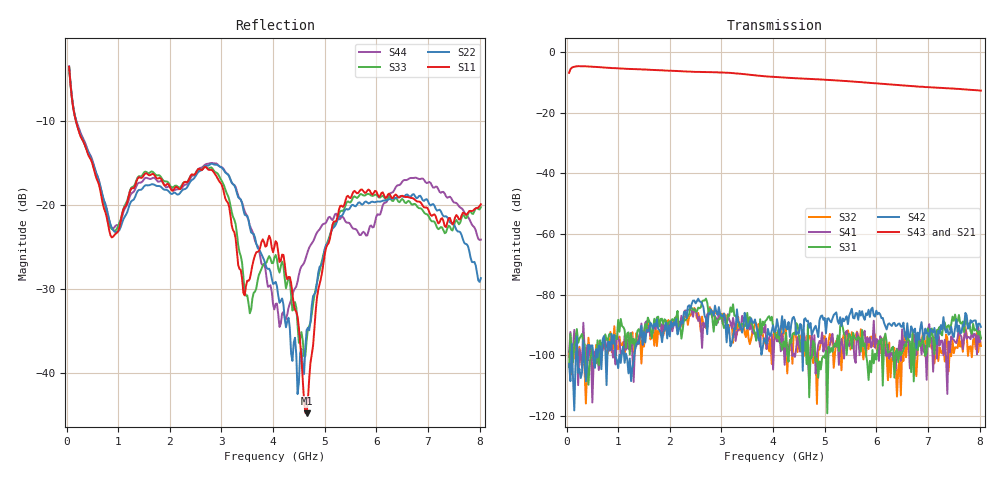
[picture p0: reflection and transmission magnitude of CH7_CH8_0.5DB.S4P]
!Agilent Technologies,E5071C,MY46316741,A.11.02
!Date: Mon Jun 01 10:30:22 2026
!Data & Calibration Information:
!1:CH7 INPUT 2:CH7 OUTPUT 3:CH8 INPUT 4:CH8 OUTPUT
!Freq	S11:SOLT4(ON)	S12:SOLT4(ON)	S13:SOLT4(ON)	S14:SOLT4(ON)
!	S21:SOLT4(ON)	S22:SOLT4(ON)	S23:SOLT4(ON)	S24:SOLT4(ON)
!	S31:SOLT4(ON)	S32:SOLT4(ON)	S33:SOLT4(ON)	S34:SOLT4(ON)
!	S41:SOLT4(ON)	S42:SOLT4(ON)	S43:SOLT4(ON)	S44:SOLT4(ON)
!PortZ  Port1:50+j0  Port2:50+j0  Port3:50+j0  Port4:50+j0
!Above PortZ is port z conversion or system Z0 setting when saving the data.
!When reading, reference impedance value at option line is always used.
# Hz S dB R 50
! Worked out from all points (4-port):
!   320 points, 50 MHz to 8.025 GHz, reference 50 ohm
!   strongest paths, dB at 50 MHz, 2.05 GHz, 4.05 GHz, 6.05 GHz, 8.025 GHz:
!     S43: -6.9, -6.2, -8.3, -10.4, -12.7
!     S21: -7.0, -6.3, -8.5, -10.6, -12.9
!     S42: -102.8, -90.6, -92.0, -85.9, -90.6
!     S31: -103.8, -88.0, -93.5, -95.2, -94.5
!     S41: -98.8, -92.0, -93.0, -101.8, -94.1
!     S32: -98.9, -89.7, -93.5, -95.8, -96.9
!   lowest |S11| = -44.8 dB at 4.65 GHz (marker M1), VSWR 1.01, Z = 50.5 + j0.334 ohm
!   |S11| at or under -10 dB: 183.9 MHz to end of sweep
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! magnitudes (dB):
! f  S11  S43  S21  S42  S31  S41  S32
! 50 MHz  -3.5  -6.9  -7.0  -102.8  -103.8  -98.8  -98.9
! 875 MHz  -23.8  -5.3  -5.3  -92.9  -93.7  -96.2  -98.8
! 2.825 GHz  -15.9  -6.7  -6.7  -85.9  -88.0  -87.5  -85.8
! 4.2 GHz  -25.9  -8.4  -8.6  -92.6  -95.5  -95.4  -92.9
! 4.65 GHz  -44.8  -8.8  -9.0  -88.7  -102.9  -97.5  -93.6
! 5.425 GHz  -19.0  -9.6  -9.8  -87.1  -99.8  -91.9  -95.8
! 8.025 GHz  -19.9  -12.7  -12.9  -90.6  -94.5  -94.1  -96.9
